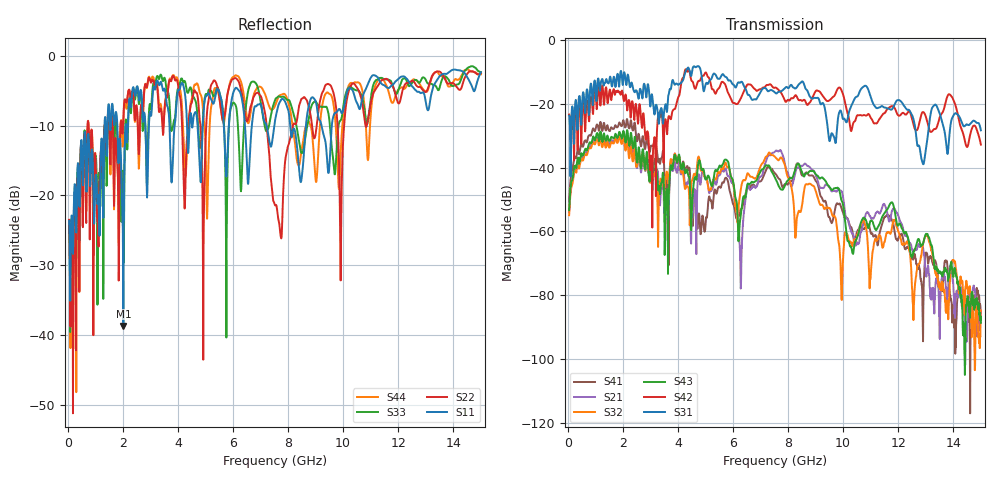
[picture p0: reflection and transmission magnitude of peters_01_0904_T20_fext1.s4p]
# MHZ S RI R 50.00
! FREQ  S11  S12  S13  S14
!  S21  S22  S23  S24
!  S31  S32  S33  S34
!  S41  S42  S43  S44
!  REAL  IMAG  REAL  IMAG  REAL  IMAG  REAL  IMAG
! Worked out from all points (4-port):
!   1496 points, 50 MHz to 15 GHz, reference 50 ohm
!   strongest paths, dB at 50 MHz, 3.79 GHz, 7.53 GHz, 11.27 GHz, 15 GHz:
!     S31: -23.7, -13.0, -16.5, -21.3, -28.3
!     S42: -23.3, -22.7, -14.9, -25.5, -32.8
!     S43: -53.4, -40.7, -43.3, -58.5, -88.6
!     S32: -54.9, -38.5, -36.7, -62.0, -84.7
!     S21: -53.9, -40.8, -34.9, -53.9, -85.1
!     S41: -50.4, -39.7, -41.8, -63.7, -85.6
!   lowest |S11| = -38.7 dB at 2.02 GHz (marker M1), VSWR 1.02, Z = 51.1 - j0.516 ohm
!   |S11| at or under -10 dB: start of sweep to 1.334 GHz; 8.078 GHz to 8.647 GHz (568.9 MHz wide, 6.8 % of centre); 9.215 GHz to 9.587 GHz (372.4 MHz wide, 3.96 % of centre)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
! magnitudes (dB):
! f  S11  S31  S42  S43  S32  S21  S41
! 50 MHz  -23.6  -23.7  -23.3  -53.4  -54.9  -53.9  -50.4
! 2.02 GHz  -38.7  -12.2  -18.4  -28.5  -30.3  -28.6  -25.1
! 3.03 GHz  -8.6  -17.9  -36.2  -40.4  -44.3  -41.1  -33.1
! 4.33 GHz  -9.9  -9.1  -9.8  -40.6  -45.7  -44.6  -39.6
! 6.28 GHz  -5.4  -13.2  -18.4  -55.1  -47.0  -77.9  -53.1
! 7.7 GHz  -6.6  -16.2  -16.0  -46.4  -37.1  -34.5  -43.7
! 15 GHz  -2.3  -28.3  -32.8  -88.6  -84.7  -85.1  -85.6
